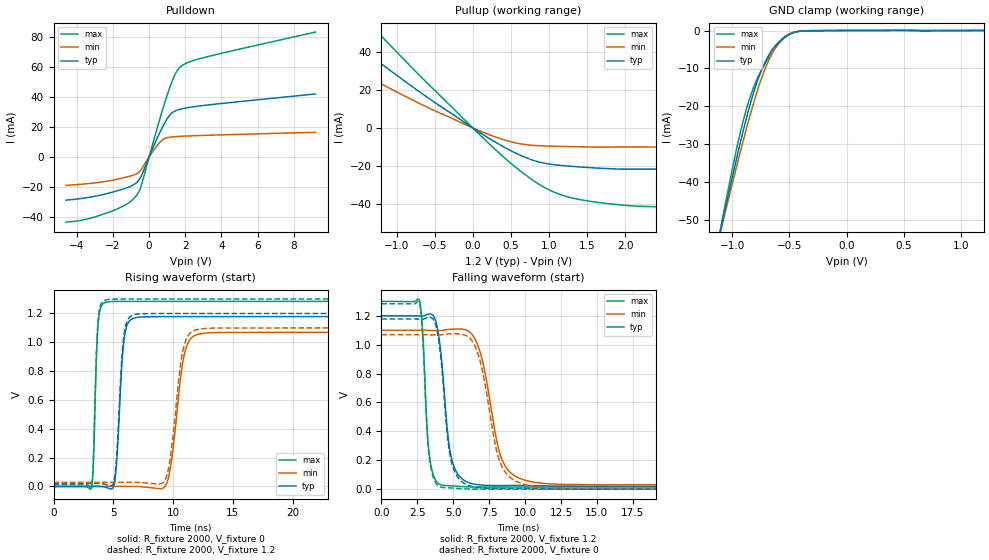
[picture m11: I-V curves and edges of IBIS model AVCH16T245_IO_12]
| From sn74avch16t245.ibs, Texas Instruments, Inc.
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[Model]   AVCH16T245_IO_12
Model_type  I/O
Vinl=0.385
Vinh=0.845
Enable   Active-Low
Vref =   0
Rref =   2000
Cref =   15p
Vmeas =   0.6
| variable   typ   min   max
C_comp   5.41pF   4.73pF   5.93pF
| C_pullup   5.89pF   3.97pF   7.93pF
| C_pulldown   5.44pF   4.83pF   7.13pF
| C_tri-state   5.41pF   4.73pF   5.93pF
[Temperature Range]   40   100   -40
| Ambient temperature   25   85   -40
[Voltage range]   1.2   1.1   1.3
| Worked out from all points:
|   slope of the pulldown table from 0 to 0.18 V, typ, clamps not added: 34.6 ohm
|   slope of the pullup table from 0 to 0.18 V, typ, clamps not added: 38.6 ohm
|   GND clamp passes 1 mA (typ) near -0.50 V on its own axis
|   rising waveform, R_fixture 2000, V_fixture 0: 20-80 % time 473ps typ, 875ps min, 285ps max; typ from 0 V to 1.18 V
|   falling waveform, R_fixture 2000, V_fixture 1.2: 20-80 % time 675ps typ, 1.22ns min, 402ps max; typ from 1.2 V to 0.02 V
|   rising waveform, R_fixture 2000, V_fixture 1.2: 20-80 % time 468ps typ, 857ps min, 283ps max; typ from 0.02 V to 1.2 V
|   falling waveform, R_fixture 2000, V_fixture 0: 20-80 % time 674ps typ, 1.22ns min, 400ps max; typ from 1.18 V to 0 V
[GND Clamp]
| AVCH16T245_IO_12
|   Voltage   I(typ)   I(min)   I(max)
-4.6V     -599.5mA   -548.1mA   -664.5mA
-1.095V   -51.65mA   -52.16mA   -51.03mA
-1.07V    -48.2mA    -49.03mA   -47.15mA
-940mV    -30.92mA   -33.24mA   -28.27mA
-840mV    -19.11mA   -21.95mA   -17.27mA
-775mV    -12.93mA   -15.39mA   -12.23mA
-695mV    -7.282mA   -8.82mA    -7.866mA
-615mV    -3.733mA   -4.168mA   -4.305mA
-545mV    -1.871mA   -1.692mA   -1.969mA
-465mV    -604.4uA   -486.8uA   -527.9uA
-355mV    -86uA      -70.97uA   -92.21uA
1.2V      714.8pA    1.474uA    -44.11nA
[Pulldown]
| AVCH16T245_IO_12
|   Voltage   I(typ)   I(min)   I(max)
-4.6V     -28.79mA   -18.92mA   -43.46mA
-3.415V   -27.06mA   -17.81mA   -41.32mA
-2.035V   -23.45mA   -15.53mA   -35.96mA
-1.17V    -20.3mA    -13.14mA   -30.86mA
-680mV    -16.87mA   -11.13mA   -25.38mA
-435mV    -12.68mA   -8.327mA   -19.06mA
440mV     12.38mA    7.543mA    19.04mA
955mV     24.67mA    12.69mA    39.57mA
1.42V     30.53mA    13.49mA    54.64mA
1.79V     32.04mA    13.78mA    60.61mA
3.17V     34.51mA    14.41mA    66.63mA
9.2V      41.96mA    16.4mA     83.17mA
[Pullup]
| AVCH16T245_IO_12
|   Voltage   I(typ)   I(min)   I(max)
-4.6V     40.24mA    7.956mA    186.3mA
-4.08V    45.4mA     8.808mA    167.8mA
-3.73V    53.62mA    9.647mA    154.2mA
-2.685V   79.31mA    16.98mA    111.4mA
-2.57V    75.87mA    21.96mA    106.5mA
-2.565V   75.72mA    49.42mA    106.3mA
-1.845V   53.66mA    37.03mA    75.82mA
-1.36V    38.76mA    26.71mA    55.3mA
575mV     -13.51mA   -7.977mA   -21.19mA
1.01V     -19.08mA   -9.527mA   -32.92mA
1.455V    -20.71mA   -9.971mA   -38.21mA
9.2V      -28.28mA   -12.48mA   -52.65mA
[Ramp]
| AVCH16T245_IO_12
| variable   typ   min   max
dV/dt_r   0.72/4.87E-10   0.65/8.93E-10   0.78/2.90E-10
dV/dt_f   0.72/6.87E-10   0.65/1.23E-09   0.78/4.15E-10
R_load = 2000
[Rising Waveform]
| AVCH16T245_IO_12
R_fixture =   2000
C_fixture =   0
L_fixture =   0
V_fixture =   0
V_fixture_min = 0
V_fixture_max = 0
|   Time   V(typ)   V(min)   V(max)
0s        18.14nV    102.1nV    431.7pV
3.16ns    600.4uV    -122.3uV   -16.25mV
3.71ns    444.3uV    150uV      1.103V
4.235ns   -2.877mV   126.9uV    1.273V
5.13ns    38.49mV    465.1uV    1.284V
5.865ns   991.1mV    360.3uV    1.284V
6.585ns   1.163V     253.7uV    1.284V
9.475ns   1.178V     21.29mV    1.284V
11.77ns   1.178V     1.046V     1.284V
29.99ns   1.178V     1.069V     1.284V
[Falling Waveform]
| AVCH16T245_IO_12
R_fixture =   2000
C_fixture =   0
L_fixture =   0
V_fixture =   1.2
V_fixture_min = 1.1
V_fixture_max = 1.3
|   Time   V(typ)   V(min)   V(max)
0s        1.2V       1.1V       1.3V
2.65ns    1.198V     1.1V       1.304V
3.315ns   1.212V     1.099V     252.3mV
4.09ns    986mV      1.098V     31.29mV
4.835ns   232.3mV    1.107V     23.43mV
6.06ns    45.58mV    1.094V     16.03mV
6.97ns    28.54mV    912.5mV    14.7mV
8.305ns   24.93mV    228.2mV    14.47mV
9.55ns    25.89mV    77.45mV    14.46mV
29.99ns   20.07mV    28.72mV    14.44mV
[Rising Waveform]
| AVCH16T245_IO_12
R_fixture =   2000
C_fixture =   0
L_fixture =   0
V_fixture =   1.2
V_fixture_min = 1.1
V_fixture_max = 1.3
|   Time   V(typ)   V(min)   V(max)
0s        20.07mV    28.66mV    14.44mV
3.155ns   20.64mV    28.59mV    -1.929mV
3.7ns     20.4mV     28.86mV    1.117V
4.225ns   17.26mV    28.81mV    1.289V
5.1ns     54.55mV    29.04mV    1.3V
5.835ns   1.01V      28.81mV    1.3V
6.555ns   1.185V     28.6mV     1.3V
9.405ns   1.2V       57.09mV    1.3V
11.64ns   1.2V       1.077V     1.3V
29.99ns   1.2V       1.1V       1.3V
[Falling Waveform]
| AVCH16T245_IO_12
R_fixture =   2000
C_fixture =   0
L_fixture =   0
V_fixture =   0
V_fixture_min = 0
V_fixture_max = 0
|   Time   V(typ)   V(min)   V(max)
0s        1.178V     1.069V     1.284V
2.65ns    1.177V     1.069V     1.287V
3.31ns    1.189V     1.069V     237.4mV
4.07ns    968.4mV    1.068V     16.93mV
4.815ns   213.5mV    1.076V     8.664mV
6.05ns    25.94mV    1.054V     1.358mV
6.895ns   9.124mV    877.4mV    245uV
8.205ns   4.983mV    201.5mV    30.45uV
9.5ns     5.791mV    48.4mV     10.42uV
29.99ns   714nV      40.7uV     185.2nV
